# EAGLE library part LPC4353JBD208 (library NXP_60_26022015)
32-bit ARM Cortex-M4/M0 MCU; up to 1 MB flash and 136 kB SRAM; Ethernet, two High-speed USB, LCD, EMC The LPC435x/3x/2x/1x are ARM Cortex-M4 based microcontrollers for embedded applications which include an ARM Cortex-M0 coprocessor, up to 1 MB of flash and 136 kB of on-chip SRAM, 16 kB of EEPROM memory, a quad SPI Flash Interface (SPIFI), advanced configurable peripherals such as the State Configurable Timer (SCT) and the Serial General Purpose I/O (SGPIO) interface, two High-speed USB controllers, Ethernet, LCD, an external memory controller, and multiple digital and analog peripherals. The LPC435x/3x/2x/1x operate at CPU frequencies of up to 204 MHz. The ARM Cortex-M4 is a next generation 32-bit core that offers system enhancements such as low power consumption, enhanced debug features, and a high level of support block integration. The ARM Cortex-M4 CPU incorporates a 3-stage pipeline, uses a Harvard architecture with separate local instruction and data buses as well as a third bus for peripherals, and includes an internal prefetch unit that supports speculative branching. The ARM Cortex-M4 supports single-cycle digital signal processing and SIMD instructions. A hardware floating-point unit is integrated in the core. The ARM Cortex-M0 coprocessor is an energy-efficient and easy-to-use 32-bit core which is upward code- and tool-compatible with the Cortex-M4 core. The Cortex-M0 coprocessor, designed as a replacement for existing 8/16-bit microcontrollers, offers up to 204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
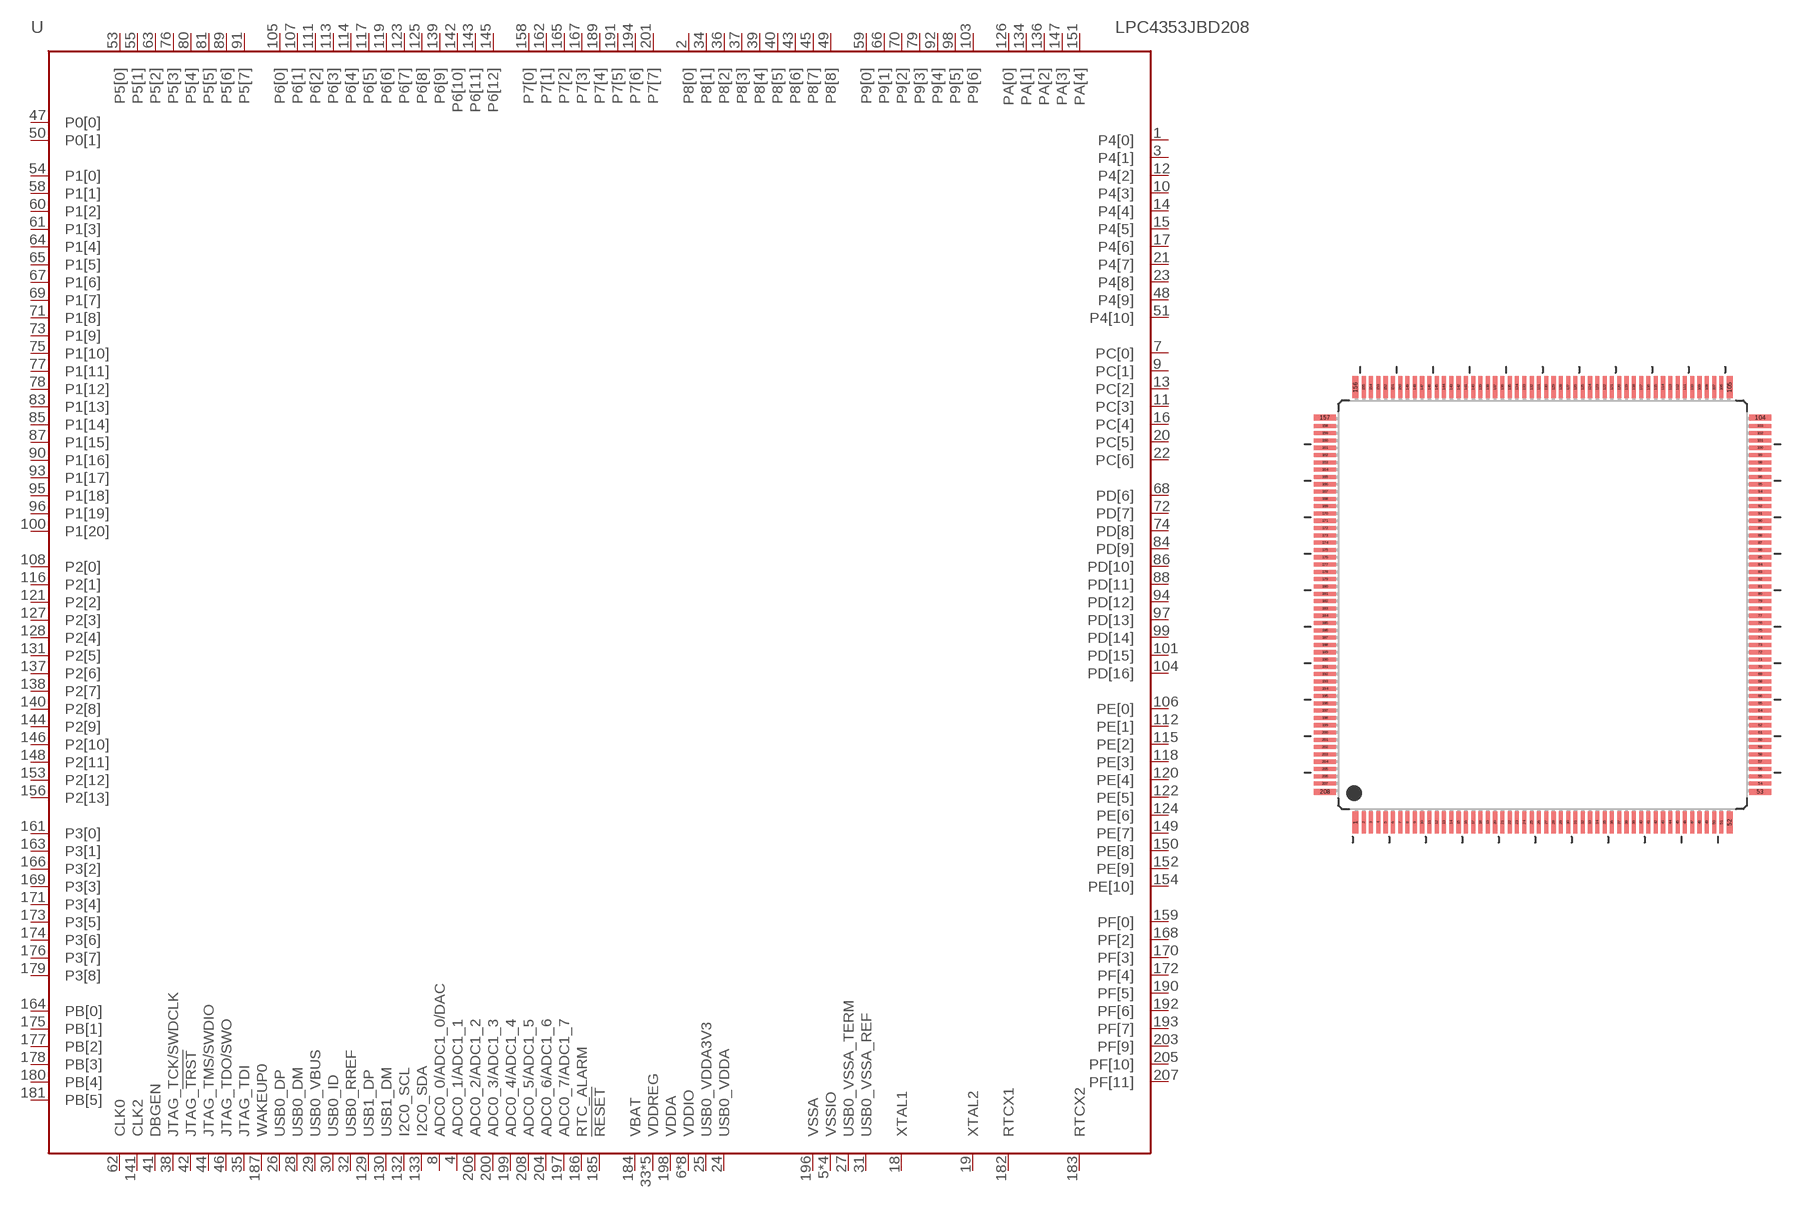
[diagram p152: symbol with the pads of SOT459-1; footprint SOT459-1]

Designator prefix U

## LPC4353JBD208  [SOT459-1]
1  P4[0]
2  P8[0]
3  P4[1]
4  ADC0_1/ADC1_1  in
5  VSSIO  pwr
6  VDDIO  pwr
7  PC[0]
8  ADC0_0/ADC1_0/DAC  in
9  PC[1]
10  P4[3]
11  PC[3]
12  P4[2]
13  PC[2]
14  P4[4]
15  P4[5]
16  PC[4]
17  P4[6]
18  XTAL1  in
19  XTAL2  out
20  PC[5]
21  P4[7]
22  PC[6]
23  P4[8]
24  USB0_VDDA  pwr
25  USB0_VDDA3V3  pwr
26  USB0_DP
27  USB0_VSSA_TERM  pwr
28  USB0_DM
29  USB0_VBUS
30  USB0_ID  in
31  USB0_VSSA_REF  pwr
32  USB0_RREF  pas
33  VDDREG  pwr
34  P8[1]
35  JTAG_TDI  in
36  P8[2]
37  P8[3]
38  JTAG_TCK/SWDCLK  in
39  P8[4]
40  P8[5]
41  DBGEN  in
42  JTAG_!TRST  in
43  P8[6]
44  JTAG_TMS/SWDIO  in
45  P8[7]
46  JTAG_TDO/SWO  out
47  P0[0]
48  P4[9]
49  P8[8]
50  P0[1]
51  P4[10]
52  VDDIO  pwr
53  P5[0]
54  P1[0]
55  P5[1]
56  VSSIO  pwr
57  VDDIO  pwr
58  P1[1]
59  P9[0]
60  P1[2]
61  P1[3]
62  CLK0
63  P5[2]
64  P1[4]
65  P1[5]
66  P9[1]
67  P1[6]
68  PD[6]
69  P1[7]
70  P9[2]
71  P1[8]
72  PD[7]
73  P1[9]
74  PD[8]
75  P1[10]
76  P5[3]
77  P1[11]
78  P1[12]
79  P9[3]
80  P5[4]
81  P5[5]
82  VDDREG  pwr
83  P1[13]
84  PD[9]
85  P1[14]
86  PD[10]
87  P1[15]
88  PD[11]
89  P5[6]
90  P1[16]
91  P5[7]
92  P9[4]
93  P1[17]
94  PD[12]
95  P1[18]
96  P1[19]
97  PD[13]
98  P9[5]
99  PD[14]
100  P1[20]
101  PD[15]
102  VDDIO  pwr
103  P9[6]
104  PD[16]
105  P6[0]
106  PE[0]
107  P6[1]
108  P2[0]
109  VSSIO  pwr
110  VDDIO  pwr
111  P6[2]
112  PE[1]
113  P6[3]
114  P6[4]
115  PE[2]
116  P2[1]
117  P6[5]
118  PE[3]
119  P6[6]
120  PE[4]
121  P2[2]
122  PE[5]
123  P6[7]
124  PE[6]
125  P6[8]
126  PA[0]
127  P2[3]
128  P2[4]
129  USB1_DP
130  USB1_DM
131  P2[5]
132  I2C0_SCL
133  I2C0_SDA
134  PA[1]
135  VDDREG  pwr
136  PA[2]
137  P2[6]
138  P2[7]
139  P6[9]
140  P2[8]
141  CLK2
142  P6[10]
143  P6[11]
144  P2[9]
145  P6[12]
146  P2[10]
147  PA[3]
148  P2[11]
149  PE[7]
150  PE[8]
151  PA[4]
152  PE[9]
153  P2[12]
154  PE[10]
155  VDDIO  pwr
156  P2[13]
157  VSSIO  pwr
158  P7[0]
159  PF[0]
160  VDDIO  pwr
161  P3[0]
162  P7[1]
163  P3[1]
164  PB[0]
165  P7[2]
166  P3[2]
167  P7[3]
168  PF[2]
169  P3[3]
170  PF[3]
171  P3[4]
172  PF[4]
173  P3[5]
174  P3[6]
175  PB[1]
176  P3[7]
177  PB[2]
178  PB[3]
179  P3[8]
180  PB[4]
181  PB[5]
182  RTCX1  in
183  RTCX2  out
184  VBAT  pwr
185  !RESET!  in
186  RTC_ALARM  out
187  WAKEUP0  in
188  VDDREG  pwr
189  P7[4]
190  PF[5]
191  P7[5]
192  PF[6]
193  PF[7]
194  P7[6]
195  VDDREG  pwr
196  VSSA  pwr
197  ADC0_7/ADC1_7  in
198  VDDA  pwr
199  ADC0_4/ADC1_4  in
200  ADC0_3/ADC1_3  in
201  P7[7]
202  VDDIO  pwr
203  PF[9]
204  ADC0_6/ADC1_6  in
205  PF[10]
206  ADC0_2/ADC1_2  in
207  PF[11]
208  ADC0_5/ADC1_5  in

## Footprint SOT459-1 (pad centres in mm)
SOT459-1 LQFP208; plastic low profile quad flat package; 208 leads; body 28 x 28 x 1.4 mm JEDEC: MS-026 IEC: 136E30 JEITA: --
smd 0.4 x 1.5: 1 -12.81,-14.9; 52 12.81,-14.9; 105 12.81,14.9; 156 -12.81,14.9
smd 0.28 x 1.5: 2 -12.25,-14.9; 3 -11.75,-14.9; 4 -11.25,-14.9; 5 -10.75,-14.9; 6 -10.25,-14.9; 7 -9.75,-14.9; 8 -9.25,-14.9; 9 -8.75,-14.9; 10 -8.25,-14.9; 11 -7.75,-14.9; 12 -7.25,-14.9; 13 -6.75,-14.9; 14 -6.25,-14.9; 15 -5.75,-14.9; 16 -5.25,-14.9; 17 -4.75,-14.9; 18 -4.25,-14.9; 19 -3.75,-14.9; 20 -3.25,-14.9; 21 -2.75,-14.9; 22 -2.25,-14.9; 23 -1.75,-14.9; 24 -1.25,-14.9; 25 -0.75,-14.9; 26 -0.25,-14.9; 27 0.25,-14.9; 28 0.75,-14.9; 29 1.25,-14.9; 30 1.75,-14.9; 31 2.25,-14.9; 32 2.75,-14.9; 33 3.25,-14.9; 34 3.75,-14.9; 35 4.25,-14.9; 36 4.75,-14.9; 37 5.25,-14.9; 38 5.75,-14.9; 39 6.25,-14.9; 40 6.75,-14.9; 41 7.25,-14.9; 42 7.75,-14.9; 43 8.25,-14.9; 44 8.75,-14.9; 45 9.25,-14.9; 46 9.75,-14.9; 47 10.25,-14.9; 48 10.75,-14.9; 49 11.25,-14.9; 50 11.75,-14.9; 51 12.25,-14.9; 106 12.25,14.9; 107 11.75,14.9; 108 11.25,14.9; 109 10.75,14.9; 110 10.25,14.9; 111 9.75,14.9; 112 9.25,14.9; 113 8.75,14.9; 114 8.25,14.9; 115 7.75,14.9; 116 7.25,14.9; 117 6.75,14.9; 118 6.25,14.9; 119 5.75,14.9; 120 5.25,14.9; 121 4.75,14.9; 122 4.25,14.9; 123 3.75,14.9; 124 3.25,14.9; 125 2.75,14.9; 126 2.25,14.9; 127 1.75,14.9; 128 1.25,14.9; 129 0.75,14.9; 130 0.25,14.9; 131 -0.25,14.9; 132 -0.75,14.9; 133 -1.25,14.9; 134 -1.75,14.9; 135 -2.25,14.9; 136 -2.75,14.9; 137 -3.25,14.9; 138 -3.75,14.9; 139 -4.25,14.9; 140 -4.75,14.9; 141 -5.25,14.9; 142 -5.75,14.9; 143 -6.25,14.9; 144 -6.75,14.9; 145 -7.25,14.9; 146 -7.75,14.9; 147 -8.25,14.9; 148 -8.75,14.9; 149 -9.25,14.9; 150 -9.75,14.9; 151 -10.25,14.9; 152 -10.75,14.9; 153 -11.25,14.9; 154 -11.75,14.9; 155 -12.25,14.9
smd 1.5 x 0.4: 53 14.9,-12.81; 104 14.9,12.81; 157 -14.9,12.81; 208 -14.9,-12.81
smd 1.5 x 0.28: 54 14.9,-12.25; 55 14.9,-11.75; 56 14.9,-11.25; 57 14.9,-10.75; 58 14.9,-10.25; 59 14.9,-9.75; 60 14.9,-9.25; 61 14.9,-8.75; 62 14.9,-8.25; 63 14.9,-7.75; 64 14.9,-7.25; 65 14.9,-6.75; 66 14.9,-6.25; 67 14.9,-5.75; 68 14.9,-5.25; 69 14.9,-4.75; 70 14.9,-4.25; 71 14.9,-3.75; 72 14.9,-3.25; 73 14.9,-2.75; 74 14.9,-2.25; 75 14.9,-1.75; 76 14.9,-1.25; 77 14.9,-0.75; 78 14.9,-0.25; 79 14.9,0.25; 80 14.9,0.75; 81 14.9,1.25; 82 14.9,1.75; 83 14.9,2.25; 84 14.9,2.75; 85 14.9,3.25; 86 14.9,3.75; 87 14.9,4.25; 88 14.9,4.75; 89 14.9,5.25; 90 14.9,5.75; 91 14.9,6.25; 92 14.9,6.75; 93 14.9,7.25; 94 14.9,7.75; 95 14.9,8.25; 96 14.9,8.75; 97 14.9,9.25; 98 14.9,9.75; 99 14.9,10.25; 100 14.9,10.75; 101 14.9,11.25; 102 14.9,11.75; 103 14.9,12.25; 158 -14.9,12.25; 159 -14.9,11.75; 160 -14.9,11.25; 161 -14.9,10.75; 162 -14.9,10.25; 163 -14.9,9.75; 164 -14.9,9.25; 165 -14.9,8.75; 166 -14.9,8.25; 167 -14.9,7.75; 168 -14.9,7.25; 169 -14.9,6.75; 170 -14.9,6.25; 171 -14.9,5.75; 172 -14.9,5.25; 173 -14.9,4.75; 174 -14.9,4.25; 175 -14.9,3.75; 176 -14.9,3.25; 177 -14.9,2.75; 178 -14.9,2.25; 179 -14.9,1.75; 180 -14.9,1.25; 181 -14.9,0.75; 182 -14.9,0.25; 183 -14.9,-0.25; 184 -14.9,-0.75; 185 -14.9,-1.25; 186 -14.9,-1.75; 187 -14.9,-2.25; 188 -14.9,-2.75; 189 -14.9,-3.25; 190 -14.9,-3.75; 191 -14.9,-4.25; 192 -14.9,-4.75; 193 -14.9,-5.25; 194 -14.9,-5.75; 195 -14.9,-6.25; 196 -14.9,-6.75; 197 -14.9,-7.25; 198 -14.9,-7.75; 199 -14.9,-8.25; 200 -14.9,-8.75; 201 -14.9,-9.25; 202 -14.9,-9.75; 203 -14.9,-10.25; 204 -14.9,-10.75; 205 -14.9,-11.25; 206 -14.9,-11.75; 207 -14.9,-12.25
